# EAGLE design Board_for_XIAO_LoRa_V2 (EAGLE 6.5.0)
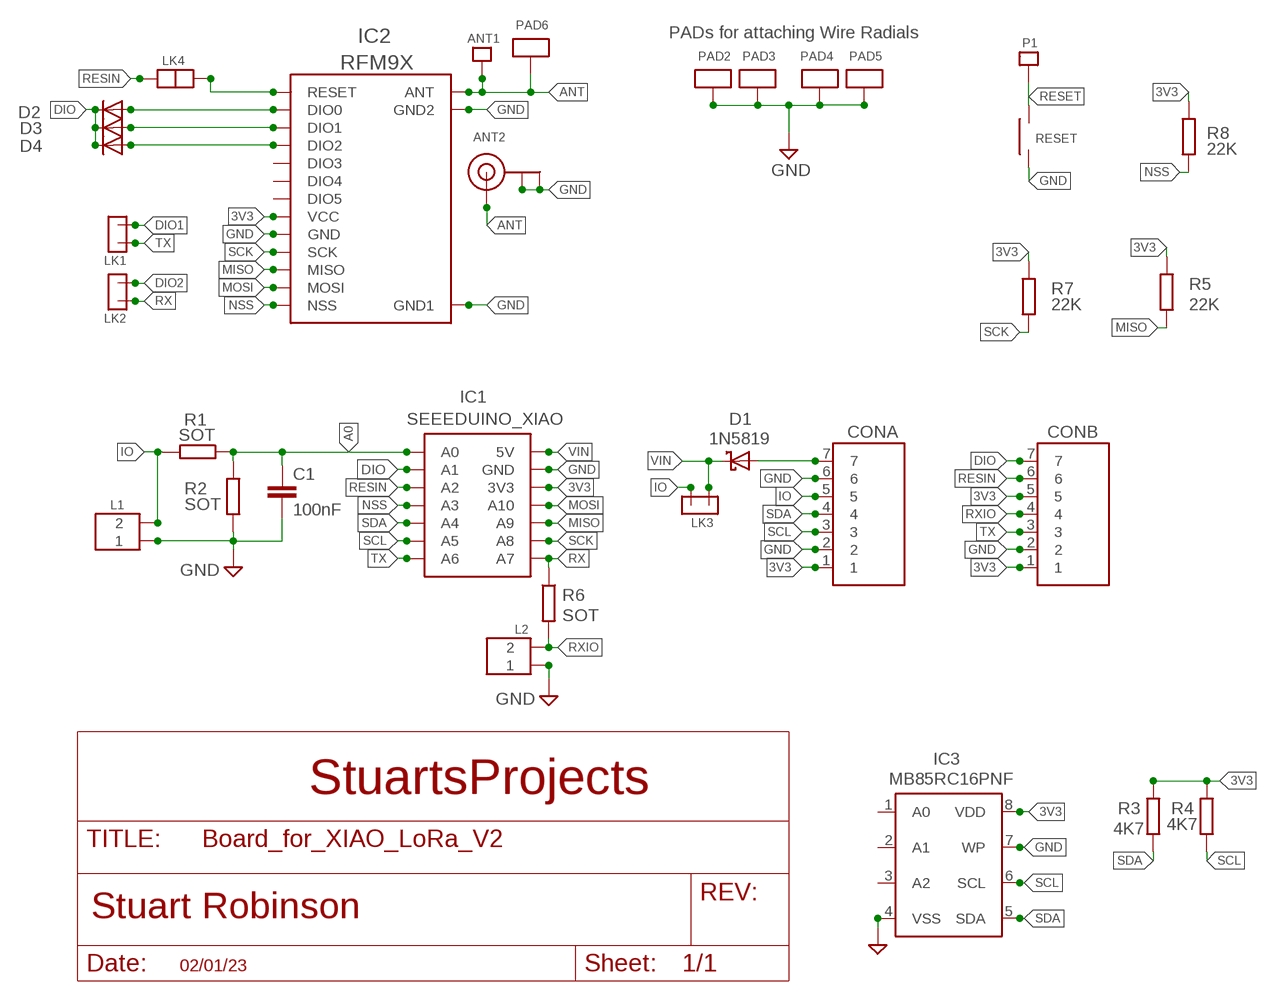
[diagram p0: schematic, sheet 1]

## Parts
ANT1  SINGLEPAD  [SINGLEPAD]
ANT2  ANTENNA_U.FL  [U.FL]
C1  100nF  AXIAL_CERAMIC  [MINI_CERAMIC_DISC]
CONA  7X1  [7X1_BATPINS]
CONB  7X1STD  [7X1]
D1  1N5819  SCHOTTKY_SMALL_DEFAULT  [SCHOTTKY_SMALL]
D2  1N4148  SIGNAL_DIODE_MIN  [SIGNAL_DIODE_MIN]
D3  1N4148  SIGNAL_DIODE_MIN  [SIGNAL_DIODE_MIN]
D4  1N4148  SIGNAL_DIODE_MIN  [SIGNAL_DIODE_MIN]
IC1  SEEEDUINO_XIAO  SEEEDUINO_XIAO_SMT_DEFAULT  [SEEEDUINO_XIAO_SMT]
IC2  RFM9X  RFM98  [RFM98]
IC3  MB85RC16PNF  24L256SOIC2  [SOIC_2]
L1  2PIN  [2PIN]
L2  2PIN  [2PIN]
LK1  2PINMICROHEADER  [2PINMICROHEADER]
LK2  2PINMICROHEADER  [2PINMICROHEADER]
LK3  2PINMICROHEADER  [2PINMICROHEADER]
LK4  2PADLINKLARGE  [2PADLINKLARGE]
P1  SINGLEPAD  [SINGLEPAD]
PAD2  ANTPAD2  [ANTPAD2]
PAD3  ANTPAD2  [ANTPAD2]
PAD4  ANTPAD2  [ANTPAD2]
PAD5  ANTPAD2  [ANTPAD2]
PAD6  ANTPAD2  [ANTPAD2]
R1  SOT  125MWRESISTOR  [125MWRESISTOR_MIN]
R2  SOT  125MWRESISTOR  [125MWRESISTOR_MIN]
R3  4K7  125MWRESISTOR  [125MWRESISTOR_MIN]
R4  4K7  125MWRESISTOR  [125MWRESISTOR_MIN]
R5  22K  125MWRESISTOR  [125MWRESISTOR_MIN]
R6  SOT  125MWRESISTOR  [125MWRESISTOR_MIN]
R7  22K  125MWRESISTOR  [125MWRESISTOR_MIN]
R8  22K  125MWRESISTOR  [125MWRESISTOR_MIN]
RESET  SMTSWITCH_4_X_3  [SMTSWITCH_4_X_3]

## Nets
3V3 [POWER]: CONA.1 CONB.1 CONB.5 IC1.3V3 IC2.13(VCC) IC3.8(VDD) R3.P$1 R4.P$1 R5.P$1 R7.P$1 R8.P$1
A0: C1.1 IC1.D0(A0) R1.P$1 R2.P$1
ANT: ANT1.P$1 ANT2.3(SIGNAL) IC2.9(ANT) PAD6.P$1
DIO: CONB.7 D2.C D3.C D4.C IC1.D1(A1)
DIO1: D3.A IC2.15(DIO1) LK1.2
DIO2: D4.A IC2.16(DIO2) LK2.2
GND [POWER]: ANT2.1(GND) ANT2.2(GND) C1.2 CONA.2 CONA.6 CONB.2 IC1.GND IC2.1(GND) IC2.8(GND1) IC2.10(GND2) IC3.4(VSS) IC3.7(WP) L1.P$1 L2.P$1 PAD2.P$1 PAD3.P$1 PAD4.P$1 PAD5.P$1 R2.P$2 RESET.1
IO: CONA.5 L1.P$2 LK3.2 R1.P$2
MISO: IC1.D9(A9) IC2.2(MISO) R5.P$2
MOSI: IC1.D10(A10) IC2.3(MOSI)
N$1 [POWER]: CONA.7 D1.A
N$2: D2.A IC2.14(DIO0)
NSS: IC1.D3(A3) IC2.5(NSS) R8.P$2
RES: IC2.6(RESET) LK4.P$2
RESET: P1.P$1 RESET.2
RESIN: CONB.6 IC1.D2(A2) LK4.P$1
RX: IC1.D7(A7) LK2.1 R6.P$1
RXIO: CONB.4 L2.P$2 R6.P$2
SCK: IC1.D8(A8) IC2.4(SCK) R7.P$2
SCL: CONA.3 IC1.D5(A5) IC3.6(SCL) R4.P$2
SDA: CONA.4 IC1.D4(A4) IC3.5(SDA) R3.P$2
TX: CONB.3 IC1.D6(A6) LK1.1
VIN [POWER]: D1.C IC1.5V LK3.1
Unconnected: IC2.7(DIO5) IC2.11(DIO3) IC2.12(DIO4) IC3.1(A0) IC3.2(A1) IC3.3(A2)

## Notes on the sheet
- PADs for attaching Wire Radials
- StuartsProjects
- 02/01/23

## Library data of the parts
ANT1 P1 = LMA2:SINGLEPAD
ANT2 = adafruit:ANTENNA_U.FL: U.FL Antenna Connector
C1 = LMA2:AXIAL_CERAMIC
CONA CONB = My_Pin_Headers:7X1
D1 = LMA2:SCHOTTKY_SMALL
D2-D4 = LMA2:SIGNAL_DIODE_MIN
IC1 = LMA2:SEEEDUINO_XIAO_SMT
IC2 = LMA2:RFM98
IC3 = LMA2:24L256
L1 L2 = LMA2:2PIN
LK1-LK3 = LMA2:2PINMICROHEADER
LK4 = LMA2:2PADLINKLARGE
PAD2-PAD6 = LMA2:ANTPAD2
R1-R8 = LMA2:125MWRESISTOR
RESET = LMA2:SMTSWITCH_4_X_3

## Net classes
0 default: width 0.203 mm
1 POWER: width 0.635 mm
2 VDD: width 0.635 mm
3 gpspower: width 0.635 mm

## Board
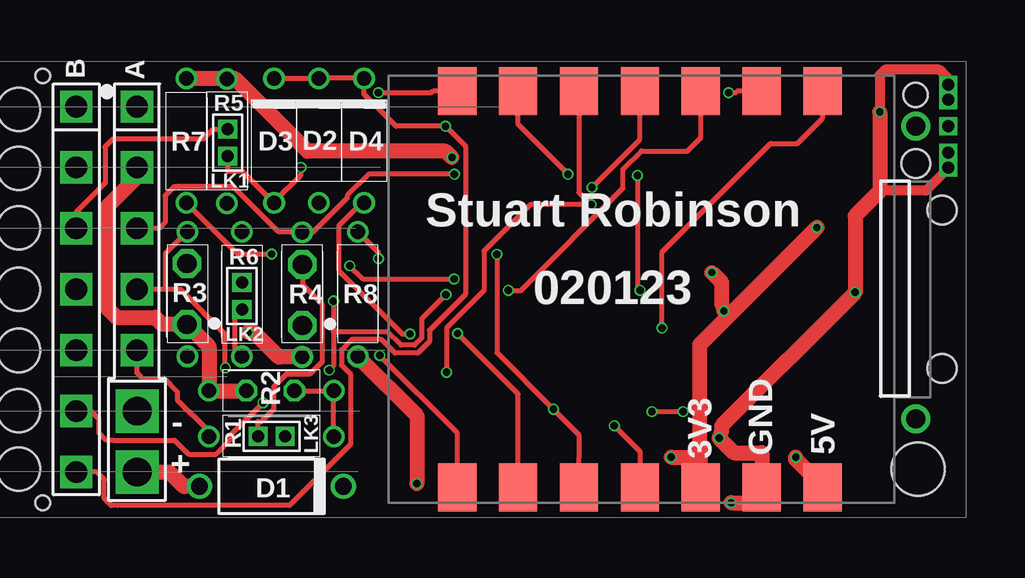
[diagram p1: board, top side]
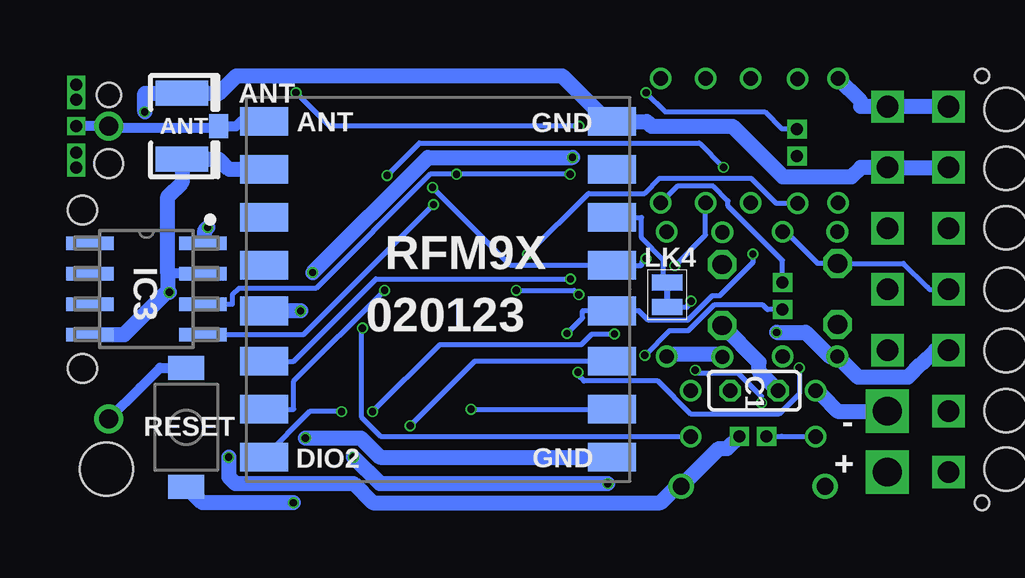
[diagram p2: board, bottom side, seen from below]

No outline drawn. Coordinates in mm, seen from the top.
Copper layers (1*16): Top 0.035559375mm / dielectric 1.6mm / Bottom 0.035559375mm
Design rules "jlcpcb2layer *": minimum track width 5mil, minimum drill 12mil, track to track 5mil, track to pad 5mil, pad to pad 5mil, via to via 5mil, smd to smd 5mil, copper to edge 8mil, drill to drill 6mil, minimum pad ring 5mil, minimum via ring 3mil, stop-mask expansion 2.5mil, vias tented up to drill 1000mil, thermal gap 10mil
Holes 1.8 mm at 1.5,14.55 1.5,12.06 1.5,9.5 1.5,6.95 1.5,4.44 1.5,2 1.5,17
Holes 1.2 mm at 38.9,14.74 40,12.8 40,6.2
Holes 2.2 mm at 39,2
Holes 1 mm at 38.9,17.6
Holes 0.6 mm at 2.5,18.4 2.5,0.6

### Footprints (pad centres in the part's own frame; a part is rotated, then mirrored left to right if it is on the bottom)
SINGLEPAD = drill 0.8: P$1 0,0
U.FL = smd 2.2 x 1.05: 1 0,1.375; 2 0,-1.375 | smd 0.8 x 1: 3 1.525,0
MINI_CERAMIC_DISC = drill 0.6 octagon: 1 -1,0; 2 1,0
7X1_BATPINS = drill 0.9 square: 1 -7.62,0; 2 -5.08,0; 3 -2.54,0; 4 0,0; 5 2.54,0 | drill 1.2 square: 6 5.08,0; 7 7.62,0
7X1 = drill 0.9 square: 1 -7.62,0; 2 -5.08,0; 3 -2.54,0; 4 0,0; 5 2.54,0; 6 5.08,0; 7 7.62,0
SCHOTTKY_SMALL = drill 0.7: A -3,0; C 3,0
SIGNAL_DIODE_MIN = drill 0.6: A -2.6,0; C 2.6,0
SEEEDUINO_XIAO_SMT = smd 2 x 1.6: 3V3 8.255,2.54; 5V 8.255,7.62; D0 -8.255,7.62; D1 -8.255,5.08; D2 -8.255,2.54; D3 -8.255,0; D4 -8.255,-2.54; D5 -8.255,-5.08; D6 -8.255,-7.62; D7 8.255,-7.62; D8 8.255,-5.08; D9 8.255,-2.54; D10 8.255,0; GND 8.255,5.08
RFM98 = smd 2 x 1.2: 1 -7.25,7; 2 -7.25,5; 3 -7.25,3; 4 -7.25,0.9; 5 -7.25,-1; 6 -7.25,-3; 7 -7.25,-5; 8 -7.25,-7; 9 7.25,-7; 10 7.25,-5; 11 7.25,-3; 12 7.25,-1; 13 7.25,0.9; 14 7.25,3; 15 7.25,5; 16 7.25,7
SOIC_2 = smd 1.981 x 0.559: 1 -2.362,1.905; 2 -2.362,0.635; 3 -2.362,-0.635; 4 -2.362,-1.905; 5 2.362,-1.905; 6 2.362,-0.635; 7 2.362,0.635; 8 2.362,1.905
2PIN = drill 0.8 octagon: P$1 0,1.27; P$2 0,-1.27
2PINMICROHEADER = drill 0.5 pad 0.8 square: 1 -0.06,0.575; 2 -0.06,-0.56
2PADLINKLARGE = smd 1.27 x 0.66: P$1 0,0.46; P$2 0,-0.56
ANTPAD2 = drill 0.5 square: P$1 0,0
125MWRESISTOR_MIN = drill 0.6: P$1 -2.6,0; P$2 2.6,0
SMTSWITCH_4_X_3 = smd 1 x 1.5: 1 -2.48,0; 2 2.48,0

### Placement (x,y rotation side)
ANT1  38.9,16.3 0 top
ANT2  35.85,16.3 0 bottom
C1  11.99,5.27 0 bottom
CONA  6.44,9.5 270 top
CONB  3.9,9.5 270 top
D1  12.04,1.28 0 top
D2  14.02,15.7 90 top
D3  12.15,15.7 90 top
D4  15.9,15.7 90 top
IC1  27.4,9.5 270 top
IC2  25.17,9.5 180 bottom
IC3  37.33,9.52 0 bottom
L1  13.33,9.26 180 top
L2  8.52,9.31 180 top
LK1  10.27,15.61 0 top
LK2  10.75,9.23 180 top
LK3  12.04,3.31 270 top
LK4  15.63,9.23 180 bottom
P1  38.9,4.1 0 top
PAD2  40.25,17.4 0 top
PAD3  40.25,18.03 0 top
PAD4  40.25,14.57 0 top
PAD5  40.25,15.2 0 top
PAD6  40.25,16.3 0 top
R1  12.04,3.35 180 top
R2  12.04,5.27 180 top
R3  8.53,9.3 90 top
R4  13.32,9.28 90 top
R5  10.19,15.68 270 top
R6  10.81,9.3 90 top
R7  8.5,15.7 270 top
R8  15.64,9.3 90 top
RESET  35.67,3.75 90 bottom

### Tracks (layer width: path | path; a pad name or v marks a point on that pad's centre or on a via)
3V3  (via drill 0.3 pad 0.46)
  Top 0.635: R4.P$1 12.35,6.68 11.32,7.7 v11.06,7.7 | v19.57,15 19.31,15.26 13.54,15.26 10.5,18.3 R5.P$1 10.1,18.3 R7.P$1 | R8.P$1 18.1,4.24 v18.1,1.4 | 31.1,8.4 v34.78,12.08 | v28.7,2.5 29.9,2.5 | v30.4,10.2 30.8,9.8 30.8,8.9 v30.9,8.6 31.1,8.4 | 29.9,2.5 29.9,1.3 IC1.3V3 | 29.9,2.5 29.9,7.2 31.1,8.4
  Bottom 0.635: v11.06,7.7 9.84,7.7 8.84,6.7 R3.P$1 7.67,5.84 5.58,5.84 5.02,6.4 5.01,6.4 4.45,6.96 CONB.5 | R7.P$1 7.56,17.36 7.56,17.12 CONA.1 CONB.1 | R8.P$1 15.54,6.8 13.5,6.8 13.4,6.7 R4.P$1 | v30.4,10.2 25.6,15 v19.57,15 | IC3.8 34.9,11.5 34.9,11.96 v34.78,12.08 | v28.7,2.5 27.6,1.4 v18.1,1.4 | v30.9,8.6 IC2.13
A0  (via drill 0.3 pad 0.46)
  Top 0.203: v28.32,7.88 28.32,11.06 32.84,15.58 33.96,15.58 35.02,16.64 IC1.D0 | R1.P$1 R2.P$1 C1.1
  Bottom 0.203: R1.P$1 27.55,3.35 28.36,4.16 28.36,7.85 v28.32,7.88
ANT
  Bottom 0.203: 34.4,16.3 ANT2.3 | 32.5,16.5 IC2.9
  Bottom 0.406: ANT2.3 33.59,16.3 33.4,16.5 32.5,16.5 | PAD6.P$1 ANT1.P$1 38.83,16.23 34.47,16.23 34.4,16.3
DIO  (via drill 0.3 pad 0.46)
  Top 0.203: IC1.D1 31.45,17.75 31.4,17.7 v31.1,17.7 | D3.C D2.C D4.C 15.9,17.64 17.24,16.3 v19.3,16.3 20.12,15.47 20.12,9.29 18.63,7.79 18.63,7.32 18.15,6.84 17.19,6.84 16.63,7.4 15.38,7.4 14.96,6.98 14.96,6.34 15.34,5.96 15.34,3.04 12.79,0.49 5.63,0.49 5.36,0.49 5.07,0.78 5.07,1.57 4.76,1.88 CONB.7
  Bottom 0.203: v19.3,16.3 29.7,16.3 v31.1,17.7
DIO1  (via drill 0.3 pad 0.46)
  Top 0.203: LK1.2 10.21,14.42 10.83,14.42 D3.A 12.2,13.2 13.27,14.27 v13.27,14.59 | v27.3,14.25 27.3,9.56 v27.41,9.46
  Bottom 0.203: IC2.15 31.19,4.5 31.19,5.67 v27.41,9.46 | v27.3,14.25 25.95,15.6 14.28,15.6 v13.27,14.59
DIO2  (via drill 0.3 pad 0.46)
  Top 0.203: v27.9,4.4 v29.2,4.4 | D4.A 15.8,13.1 14.85,12.15 14.85,10.29 17.5,7.64 v17.82,7.64
  Bottom 0.203: v27.9,4.4 25.1,7.2 19.2,7.2 18.76,7.64 v17.82,7.64 | LK2.2 10.81,10.71 13.09,12.98 13.09,13.19 13.7,13.8 15.2,13.8 D4.A | v29.2,4.4 30.52,4.4 IC2.16
GND  (via drill 0.3 pad 0.46)
  Top 0.406: PAD5.P$1 PAD4.P$1 40.25,14.55 39.31,13.61 37.41,13.61 37.4,13.6 | v37.4,16.9 37.38,16.9 | PAD3.P$1 PAD2.P$1 40.25,18.3 40,18.55 39.89,18.66 37.61,18.66 37.4,18.45 v37.4,16.9 | v37.4,16.91 v37.4,16.9
  Top 0.635: C1.2 R2.P$2 9.44,7.12 L2.P$1 7.47,8.04 7.19,8.33 5.58,8.33 5.17,8.74 5.17,12.93 6.44,14.2 CONA.2 | PAD2.P$1 40.3,17.4 | v37.4,16.9 37.4,13.6 36.38,12.58 v36.38,9.38 30.8,3.8 30.8,3.6 v30.7,3.3 31.31,2.69 32.48,2.69 IC1.GND 32.4,1.2 32.4,0.6 v31.2,0.6
  Bottom 0.406: 36.44,10.15 36.29,10.15 IC3.7
  Bottom 0.635: 36.44,9.44 36.44,10.15 36.44,13.37 35.85,13.96 ANT2.2 34.3,14.93 33.88,14.5 IC2.10 | 36.44,9.44 v36.38,9.38 | 36.44,9.44 38.26,7.62 IC3.4 | CONB.2 CONA.2 7.56,14.58 7.94,14.2 10.8,14.2 12.9,16.3 16.27,16.3 16.48,16.5 IC2.8 18.2,16.6 20,18.4 33.58,18.4 34.3,17.68 ANT2.1 37.4,17.68 v37.4,16.91 v37.4,16.9 | C1.2 11.79,6.08 11.79,6.46 L1.P$1 | R2.P$2 9.2,5.1 8.52,4.42 CONA.6 | v30.7,3.3 28.4,3.3 27.6,2.5 IC2.1 | v31.2,0.6 35,0.6 RESET.1
IO
  Top 0.203: L1.P$2 13.33,9.7 14.17,8.87 14.17,6.49 13.65,5.97 12.68,5.97 12.15,5.44 12.15,4.51 11.64,4 11.48,4 LK3.2 | R1.P$2 9.44,3.58 8.12,4.9 8.12,5.23 7.56,5.79 6.66,5.79 6.6,5.85 6.44,6.01 CONA.5
  Bottom 0.203: LK3.2 10.85,3.37 10.83,3.35 R1.P$2
MISO  (via drill 0.3 pad 0.46)
  Top 0.203: IC1.D9 24.86,2.47 24.86,3.44 v23.8,4.5 21.44,6.86 v21.44,10.96
  Bottom 0.203: v21.44,10.96 18.9,13.5 16.56,13.5 15.93,14.13 12.13,14.13 11.1,13.1 10.2,13.1 R5.P$2 | v23.8,4.5 IC2.2
MOSI  (via drill 0.3 pad 0.46)
  Top 0.203: v26.34,3.81 27.4,2.75 IC1.D10
  Bottom 0.203: IC2.3 23.65,6.5 v26.34,3.81
N$1
  Top 0.635: CONA.7 7.79,1.88 8.38,1.28 D1.A
N$2  (via drill 0.3 pad 0.46)
  Top 0.203: v15.3,10.48 15.86,9.93 v19.66,9.93
  Bottom 0.203: IC2.14 31.19,6.5 27.76,9.93 v19.66,9.93 | v15.3,10.48 14.02,11.77 D2.A
N$3
  Bottom 0.254: 15.62,8.82 15.62,9.83
NSS  (via drill 0.3 pad 0.46)
  Top 0.203: v25.4,13.75 27.4,15.75 IC1.D3 | v16.5,10.79 16.5,11.04 R8.P$2
  Bottom 0.203: v25.4,13.75 22.15,10.5 IC2.5 16.69,10.5 16.69,10.6 v16.5,10.79
RES
  Bottom 0.203: IC2.6 16.69,12.5 16.69,11.65 15.77,10.73 15.77,9.93 LK4.P$2
RESET
  Bottom 0.406: P1.P$1 37.6,5.4 37.59,5.4 36.76,6.23 RESET.2
RESIN  (via drill 0.3 pad 0.46)
  Top 0.203: v19.31,9.28 18.3,8.27 18.3,7.46 18.01,7.17 17.44,7.17 16.88,7.73 14.62,7.73 | 14.62,7.73 14.62,6.3 v14.45,6.13 | v14.62,9.01 14.62,7.73 | v21.91,9.46 22.45,9.46 26.7,13.72 26.7,14.52 27.45,15.27 29.39,15.27 29.94,15.82 IC1.D2 | v11.69,4.77 10.37,3.45 10.37,3.26 9.73,2.62 8.59,2.62 8,3.21 5.45,3.21 5.16,3.21 4.86,3.51 4.86,4.08 4.52,4.42 CONB.6
  Bottom 0.203: LK4.P$1 14.77,8.77 14.77,8.87 v14.62,9.01 | v21.91,9.46 19.49,9.46 v19.31,9.28 | v11.69,4.77 11.69,5.04 12.65,6 14.32,6 v14.45,6.13
RX  (via drill 0.3 pad 0.46)
  Top 0.203: LK2.1 10.52,8.36 10.52,7 R6.P$1 | v16.55,6.75 19.78,3.52 IC1.D7
  Bottom 0.203: LK2.1 11.44,8.65 11.62,8.84 13.68,8.84 14.75,7.76 15.54,7.76 v16.55,6.75
RXIO
  Bottom 0.203: R6.P$2 10.67,11.9 9.35,10.58 L2.P$2 5.77,10.58 4.8,9.61 4.69,9.5 CONB.4
SCK  (via drill 0.3 pad 0.46)
  Top 0.203: IC1.D8 22.32,5.14 v19.8,7.66 | R7.P$2 10.63,10.97 v12.05,10.97
  Bottom 0.203: v19.8,7.66 19.15,8.31 19.15,8.6 IC2.4 16.79,8.6 16.69,8.5 16.4,8.21 14.77,8.21 13.76,9.22 13.44,9.22 12.05,10.62 v12.05,10.97
SCL  (via drill 0.3 pad 0.46)
  Top 0.203: R4.P$2 12.34,11.89 10.45,13.78 8.18,13.78 7.99,13.78 7.61,13.4 7.61,12.3 7.35,12.04 CONA.3 | v19.67,14.3 16.1,14.3 15.2,13.4 15.2,13.3 13.8,11.9 13.36,11.9 R4.P$2 | R4.P$2 | v24.4,14.3 22.32,16.38 IC1.D5
  Bottom 0.203: IC3.6 33.75,8.88 33.75,9.27 33.48,9.54 30.26,9.54 25.5,14.3 v24.4,14.3 v19.67,14.3
SDA  (via drill 0.3 pad 0.46)
  Top 0.203: 7.62,9.5 CONA.4 | v10.12,6.23 10.12,7.63 8.25,9.5 7.62,9.5 | R3.P$2 7.62,10.98 7.62,9.5 | v19.34,6.04 19.34,7.9 20.9,9.46 20.9,11.09 22.84,13.04 v25.36,13.04 24.86,13.54 IC1.D4
  Bottom 0.203: v10.12,6.23 10.12,5.15 10.97,4.29 14.62,4.29 16,5.67 19.1,5.67 19.34,5.91 v19.34,6.04 | IC3.5 30.79,7.62 v25.36,13.04
TX  (via drill 0.3 pad 0.46)
  Top 0.203: IC1.D6 18.75,17.75 18.7,17.7 v16.5,17.7 | CONB.3 3.9,12.72 5.11,13.93 5.11,15.42 5.11,15.45 5.44,15.78 9.22,15.78 9.62,16.18 LK1.1
  Bottom 0.203: LK1.1 10.84,16.18 11.55,16.9 15.7,16.9 v16.5,17.7
VIN  (via drill 0.3 pad 0.46)
  Top 0.635: v33.9,2.5 33.9,2.4 35,1.3 IC1.5V
  Bottom 0.635: v33.9,2.5 33.9,1.68 33.62,1.4 28.7,1.4 27.9,0.6 15.9,0.6 15.3,1.2 D1.C 13.46,2.86 13.12,2.86 LK3.1

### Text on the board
tPlace: B | A | Stuart Robinson | 020123 | - | +
bPlace: ANT | ANT | LK4 | RFM9X | 020123 | - | +
tNames: R5 | R7 | D3 | D2 | D4 | LK1 | R6 | R3 | R4 | R8 | LK2 | R2 | R1 | LK3 | GND | 5V | D1 | 3V3
bNames: GND | ANT | IC3 | C1 | RESET | GND | DIO2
